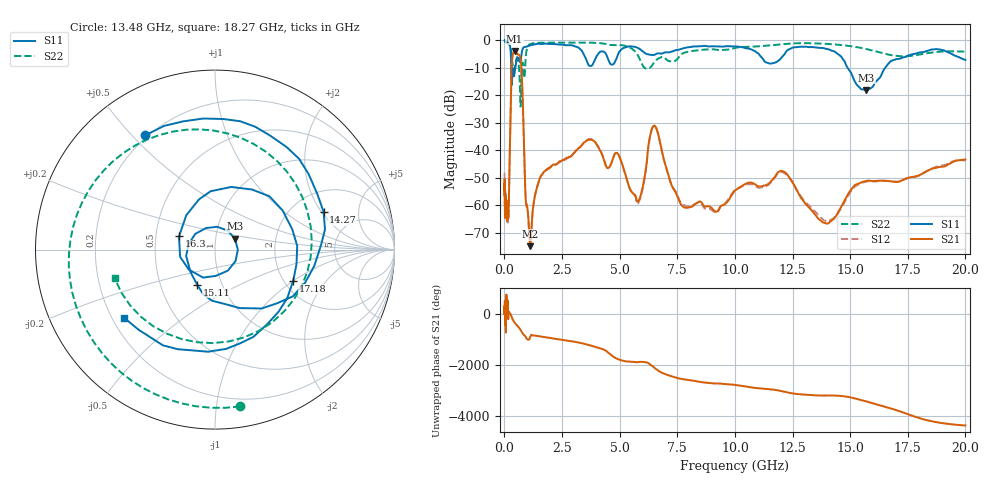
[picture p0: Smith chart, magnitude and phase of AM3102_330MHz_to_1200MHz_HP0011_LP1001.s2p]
! Date/Time: Tue, Sep 11, 2018 5:12 PM
! Network Analyzer: Agilent Technologies E8362B Rev: A.07.50.63
! Sweep from 0.010 to 20.000 GHz, 1601 Points, Sweep Type: LOG
! Power Supply: 4.949 V, 0.001 A
# Hz S DB R 50
!freq MagS11 AngS11 MagS21 AngS21 MagS12 AngS12 MagS22 AngS22
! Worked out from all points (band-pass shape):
!   1601 points, 10 MHz to 20 GHz, reference 50 ohm
!   highest |S21| = -3.84 dB at 445.1 MHz (marker M1); lowest = -74.9 dB at 1.119 GHz (marker M2)
!   |S21| within 3 dB of the highest: 334.8 MHz to 703.5 MHz (368.7 MHz wide, 71 % of centre)
!   lowest |S11| = -18.0 dB at 15.7 GHz (marker M3), VSWR 1.29, Z = 61.9 + j7.62 ohm
!   |S11| at or under -10 dB: 299 MHz to 476.2 MHz (177.2 MHz wide, 45.7 % of centre); 14.89 GHz to 16.52 GHz (1.623 GHz wide, 10.3 % of centre)
!   |S22| runs from -24.0 to -0.3 dB; largest |S21 - S12| = 0.012
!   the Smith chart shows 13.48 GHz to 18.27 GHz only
!   S11 on the Smith chart (normalised r, x): 13.48 GHz: 0.19, +0.55; 14.27 GHz: 2.95, +2.10; 15.11 GHz: 0.76, -0.31; 16.3 GHz: 0.66, +0.10; 17.18 GHz: 2.24, -1.00; 18.27 GHz: 0.25, -0.32
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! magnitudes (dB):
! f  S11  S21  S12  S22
! 10 MHz  0.0  -52.4  -48.1  -0.3
! 35.55 MHz  0.0  -63.9  -62.2  -0.5
! 126.4 MHz  -0.4  -62.5  -63.4  -1.0
! 180.5 MHz  -1.0  -62.0  -63.8  -1.3
! 313.2 MHz  -15.4  -9.8  -9.8  -5.5
! 445.1 MHz  -11.7  -3.8  -3.9  -9.9
! 447.2 MHz  -11.5  -3.8  -3.9  -9.8
! 722.6 MHz  -6.3  -8.4  -8.5  -21.4
! 1.119 GHz  -1.8  -74.9  -74.4  -1.3
! 1.59 GHz  -1.3  -49.3  -49.3  -0.8
! 3.757 GHz  -9.3  -36.0  -35.9  -0.8
! 5.652 GHz  -2.3  -56.1  -56.4  -3.8
! 6.518 GHz  -5.2  -31.0  -31.2  -7.7
! 7.845 GHz  -2.7  -60.8  -60.2  -4.4
! 13.48 GHz  -2.5  -63.4  -62.3  -1.1
! 14.27 GHz  -3.9  -65.0  -64.7  -1.4
! 15.11 GHz  -13.2  -53.5  -54.0  -2.2
! 15.7 GHz  -18.0  -51.2  -51.4  -3.1
! 16.3 GHz  -13.4  -51.0  -51.1  -4.4
! 17.18 GHz  -6.6  -51.2  -51.1  -5.7
! 18.27 GHz  -4.0  -47.8  -47.9  -4.7
! 20 GHz  -7.1  -43.3  -43.7  -4.1
